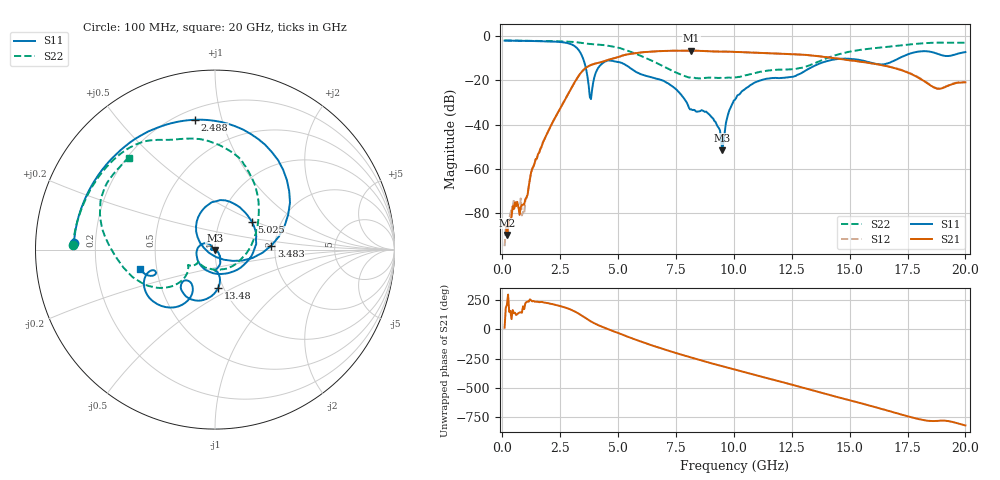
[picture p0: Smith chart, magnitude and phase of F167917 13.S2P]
!  2-Port S-parameters saved by WinCal
! VAR MeasName=S-Parameters (CALIBRATED_DATA) read from VNA (N5242A)
! VAR MeasDate=2016-11-22 9:00:19
! VAR NAME=F167917 13
! VAR FILENAME=F167917 13.S2P
! VAR DATE=2016-11-22 9:00:19
! VAR PHYS_PORTS=1,2
# Hz S DB R 50
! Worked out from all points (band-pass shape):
!   401 points, 100 MHz to 20 GHz, reference 50 ohm
!   highest |S21| = -6.59 dB at 8.159 GHz (marker M1); lowest = -89.9 dB at 199.5 MHz (marker M2)
!   |S21| within 3 dB of the highest: 4.989 GHz to 14.04 GHz (9.048 GHz wide, 95.1 % of centre)
!   lowest |S11| = -51.7 dB at 9.503 GHz (marker M3), VSWR 1.01, Z = 49.9 - j0.247 ohm
!   |S11| at or under -10 dB: 3.482 GHz to 17.15 GHz (13.66 GHz wide, 132 % of centre)
!   |S22| runs from -19.2 to -2.0 dB; largest |S21 - S12| = 0.0048
!   S11 on the Smith chart (normalised r, x): 100 MHz: 0.12, +0.02; 2.488 GHz: 0.26, +0.82; 3.483 GHz: 1.91, +0.10; 5.025 GHz: 1.43, +0.47; 13.48 GHz: 0.95, -0.42; 20 GHz: 0.40, -0.11
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1e8  -2.09 177.3  -85.62 14.1  -94.92 -28.4  -2.03 178.3
1.995e8  -2.09 174.7  -89.89 -151.2  -86.59 -173.4  -2.04 176.7
9.4575e8  -2.21 154.7  -76.15 172.5  -80.41 -156.4  -2.16 165.1
1.34375e9  -2.28 143.3  -58.96 -117.9  -59.11 -119.0  -2.23 158.9
2.488e9  -2.71 98.9  -32.97 -161.1  -32.96 -161.5  -2.43 139.3
3.43325e9  -8.79 11.6  -16.16 117.0  -16.16 117.0  -3.15 118.6
3.483e9  -10.03 4.1  -15.59 110.7  -15.57 110.6  -3.22 117.6
3.83125e9  -28.51 -150.4  -13.09 67.3  -13.06 67.1  -3.66 111.1
4.22925e9  -13.28 112.7  -11.91 28.5  -11.90 28.3  -3.97 102.1
5.02525e9  -11.81 36.7  -9.47 -32.3  -9.50 -32.6  -5.33 78.1
6.7665e9  -19.53 -168.4  -6.84 -155.9  -6.84 -156.0  -12.73 17.6
8.1595e9  -33.12 153.8  -6.59 120.1  -6.60 120.0  -18.84 -79.2
8.90575e9  -35.15 -179.6  -6.89 77.8  -6.89 77.8  -18.83 -124.4
9.50275e9  -51.69 -108.2  -7.06 46.4  -7.07 46.4  -18.98 -141.0
1.005e10  -28.76 -51.4  -7.20 17.1  -7.21 17.2  -18.73 -143.6
1.179125e10  -18.93 -92.0  -7.94 -73.3  -7.91 -73.2  -15.31 -149.5
1.338325e10  -13.98 -83.3  -8.83 -158.4  -8.79 -157.9  -12.77 -137.4
1.348275e10  -13.47 -84.9  -8.97 -163.7  -8.91 -163.4  -12.33 -137.0
1.507475e10  -10.39 -124.8  -11.07 112.9  -11.00 112.8  -6.95 -155.7
1.67165e10  -12.12 -120.0  -13.88 24.4  -13.83 24.6  -4.80 -179.8
1.875625e10  -7.91 -160.4  -23.72 -59.5  -23.56 -59.8  -3.03 149.7
2e10  -7.28 -165.5  -20.92 -97.9  -20.78 -98.4  -3.06 133.2
